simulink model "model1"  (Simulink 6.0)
settings: Solver=ode1  StartTime=0.0  StopTime=3.0  FixedStep=0.001  RelTol=1e-3
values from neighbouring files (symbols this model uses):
  a = 0.001    [slpriv1m.m]    (also in red1m.m; SAUAnalizeProject.m = axes( 'Parent',  centerPanel,   'Projection', 'perspective',; TESTm.m)
  ak0 = 1    [slpriv1m.m]    (also in TESTm.m)
  ak1 = 0.5    [slpriv1m.m]    (also in TESTm.m)
  ap0 = 1    [slpriv1m.m]    (also in TESTm.m)
  ap1 = 0.001    [slpriv1m.m]    (also in TESTm.m)
  bk0 = 0    [slpriv1m.m]    (also in TESTm.m)
  bk1 = 0.5    [slpriv1m.m]    (also in TESTm.m)
  bp0 = 1    [slpriv1m.m]    (also in TESTm.m)
  bp1 = 0.001    [slpriv1m.m]    (also in TESTm.m)
  c = 2000000    [slpriv1m.m]    (also in red1m.m; TESTm.m)
  F1 = 0    [slpriv1m.m]    (also in main5.m = peaks(35); main7.m = zeros(A1n,A2n); red1m.m; TESTm.m)
  F2 = 0    [slpriv1m.m]    (also in main5.m = membrane; main7.m = zeros(A1n,A2n); red1m.m; TESTm.m)
  G1 = 0    [slpriv1m.m]    (also in red1m.m; TESTm.m)
  G2 = 0    [slpriv1m.m]    (also in red1m.m; TESTm.m)
  i = 100    [slpriv1m.m]    (also in red1m.m; SAUAnalizeProject.m = find( isoLevel == src ); TESTm.m)
  J = 0.04    [slpriv1m.m]    (also in TESTm.m)
  Jn = 200    [slpriv1m.m]    (also in red1m.m; TESTm.m)
  k1 = 1/R    (= 2)    [myparam.m]    (also in slpriv1m.m; TESTm.m)
  K1 = 3    [dz.m]    (also in fun_F6.m = A2; fun_F7.m = A2; fun_F9.m = A1m1(i); main7.m = 0.5)
  K2 = 2    [dz.m]    (also in fun_F6.m = A1; fun_F7.m = A1; fun_F9.m = A2m1(j); main7.m = 0.5)
  K3 = 0    [dz.m]    (also in fun_F6.m = A1; fun_F7.m = A1; fun_F9.m = A3m1(k); main7.m = 0.5)
  Kc = 0.0015    [slpriv1m.m]    (also in TESTm.m)
  Ki = 0.0003    [slpriv1m.m]    (also in TESTm.m)
  Kk = 22500    [slpriv1m.m]    (also in TESTm.m)
  km = 0.36    [myparam.m]    (also in slpriv1m.m; TESTm.m)
  kv = 0.45    [myparam.m]    (also in slpriv1m.m; TESTm.m)
  T = L/R    (= 0.02)    [myparam.m]    (also in slpriv1m.m; TESTm.m)

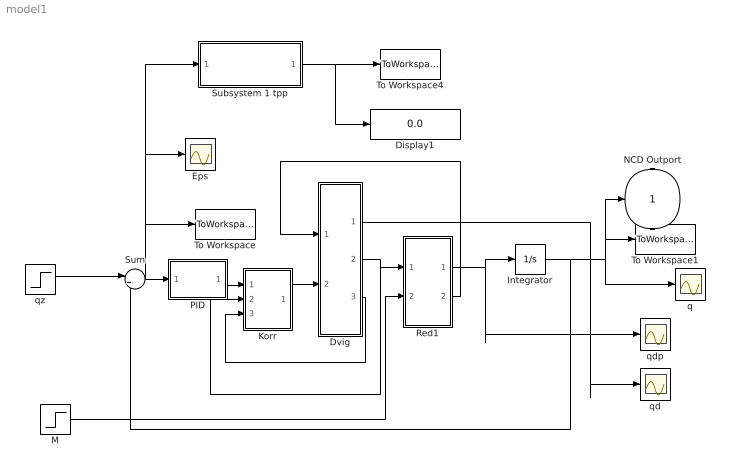
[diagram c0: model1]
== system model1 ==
  Display1 : Display
  Dvig : Subsystem  AncestorBlock=simulink3/Signals & Systems/SubSystem
  Eps : Scope
  Integrator : Integrator
  Korr : Subsystem
  M : Step  Time=0  After=0  SampleTime=0
  PID : Subsystem
  Red1 : Subsystem
  Subsystem 1 tpp : Subsystem
  Sum : Sum  Inputs=|+-
  To Workspace : ToWorkspace  VariableName=simouteps  SampleTime=-1  SaveFormat=Structure
  To Workspace1 : ToWorkspace  VariableName=simoutq  SampleTime=-1  SaveFormat=Structure
  To Workspace4 : ToWorkspace  VariableName=tpptek  SampleTime=-1  SaveFormat=Array
  q : Scope
  qd : Scope
  qdp : Scope
  qz : Step  Time=0  After=0.1  SampleTime=0
  NCD Outport : Outport  InitialOutput=0
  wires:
  Sum/1 -> PID/1(eps), To Workspace/1, Eps/1, Subsystem 1 tpp/1(In1:Signal)
  PID/1(ueps) -> Korr/1(u_eps)
  Red1/2(M2M) -> Dvig/1(Mv)
  Korr/1(u_d) -> Dvig/2(u)
  Dvig/2(qd') -> Red1/1(q1p), Korr/2(qdp)
  Dvig/3(ia) -> Korr/3(ia)
  M/1 -> Red1/2(-M2)
  Red1/1(q2p) -> Integrator/1, qdp/1
  Integrator/1 -> Sum/2, To Workspace1/1, NCD Outport/1, q/1
  Dvig/1(qd) -> qd/1
  Subsystem 1 tpp/1(Out1:tpp) -> To Workspace4/1, Display1/1
  qz/1 -> Sum/1

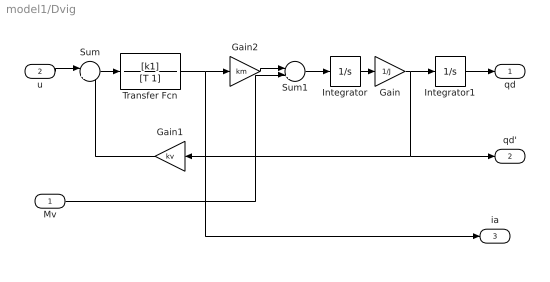
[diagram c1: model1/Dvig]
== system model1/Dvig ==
  Mv : Inport  Port=1  LatchInput=off
  u : Inport  Port=2  LatchInput=off
  Gain : Gain  Gain=1/J
  Gain1 : Gain  Orientation=left  Gain=kv
  Gain2 : Gain  Gain=km
  Integrator : Integrator
  Integrator1 : Integrator
  Sum : Sum  Inputs=|+-
  Sum1 : Sum  Inputs=|++
  Transfer Fcn : TransferFcn  Numerator=[k1]  Denominator=[T 1]
  qd : Outport
  qd' : Outport  Port=2
  ia : Outport  Port=3
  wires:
  u/1 -> Sum/1
  Gain1/1 -> Sum/2
  Sum/1 -> Transfer Fcn/1
  Transfer Fcn/1 -> Gain2/1, ia/1
  Gain2/1 -> Sum1/1
  Mv/1 -> Sum1/2
  Sum1/1 -> Integrator/1
  Integrator/1 -> Gain/1
  Gain/1 -> Integrator1/1, Gain1/1, qd'/1
  Integrator1/1 -> qd/1

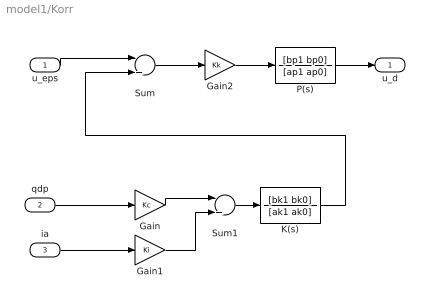
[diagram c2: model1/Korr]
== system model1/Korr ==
  u_eps : Inport  Port=1  LatchInput=off
  qdp : Inport  Port=2  LatchInput=off
  ia : Inport  Port=3  LatchInput=off
  Gain : Gain  Gain=Kc
  Gain1 : Gain  Gain=Ki
  Gain2 : Gain  Gain=Kk
  K(s) : TransferFcn  Numerator=[bk1 bk0]  Denominator=[ak1 ak0]
  P(s) : TransferFcn  Numerator=[bp1 bp0]  Denominator=[ap1 ap0]
  Sum : Sum  Inputs=|+-
  Sum1 : Sum  Inputs=|++
  u_d : Outport
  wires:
  u_eps/1 -> Sum/1
  qdp/1 -> Gain/1
  ia/1 -> Gain1/1
  Sum/1 -> Gain2/1
  Gain/1 -> Sum1/1
  Gain1/1 -> Sum1/2
  Gain2/1 -> P(s)/1
  P(s)/1 -> u_d/1
  Sum1/1 -> K(s)/1
  K(s)/1 -> Sum/2

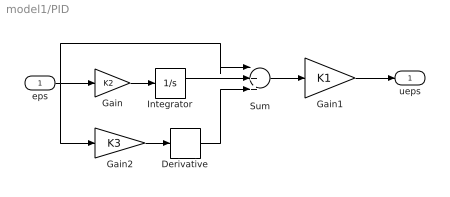
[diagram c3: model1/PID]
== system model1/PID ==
  eps : Inport  Port=1  LatchInput=off
  Derivative : Derivative
  Gain : Gain  Gain=K2
  Gain1 : Gain  Gain=K1
  Gain2 : Gain  Gain=K3
  Integrator : Integrator
  Sum : Sum  Inputs=|+++
  ueps : Outport
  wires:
  Gain1/1 -> ueps/1
  Sum/1 -> Gain1/1
  Gain/1 -> Integrator/1
  eps/1 -> Gain/1, Sum/1, Gain2/1
  Integrator/1 -> Sum/2
  Gain2/1 -> Derivative/1
  Derivative/1 -> Sum/3

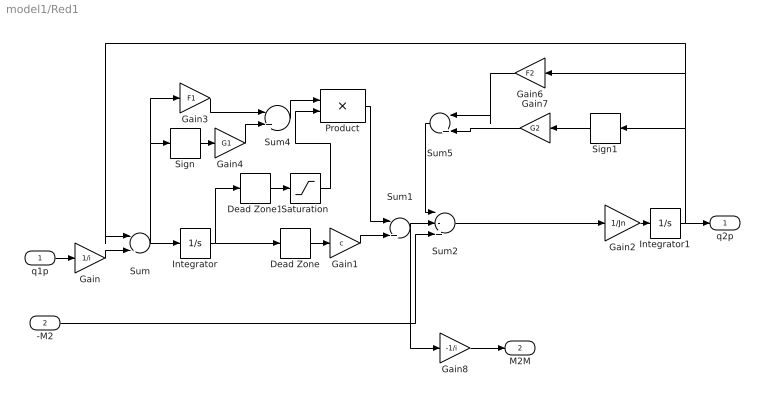
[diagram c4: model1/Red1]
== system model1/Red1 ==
  q1p : Inport  Port=1  LatchInput=off
  -M2 : Inport  Port=2  LatchInput=off
  Dead Zone : DeadZone  LowerValue=-a  UpperValue=a
  Dead Zone1 : DeadZone  LowerValue=-a  UpperValue=a
  Gain : Gain  Gain=1/i
  Gain1 : Gain  Gain=c
  Gain2 : Gain  Gain=1/Jn
  Gain3 : Gain  Gain=F1
  Gain4 : Gain  Gain=G1
  Gain6 : Gain  Orientation=left  Gain=F2
  Gain7 : Gain  Orientation=left  Gain=G2
  Gain8 : Gain  Gain=-1/i
  Integrator : Integrator
  Integrator1 : Integrator
  Product : Product
  Saturation : Saturate  UpperLimit=a  LowerLimit=-a
  Sign : Signum
  Sign1 : Signum  Orientation=left
  Sum : Sum  Inputs=|-+
  Sum1 : Sum  Inputs=|++
  Sum2 : Sum  Inputs=|-++
  Sum4 : Sum  Inputs=|++
  Sum5 : Sum  Orientation=left  Inputs=|++
  q2p : Outport
  M2M : Outport  Port=2
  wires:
  q1p/1 -> Gain/1
  Gain/1 -> Sum/2
  Sum/1 -> Integrator/1, Gain3/1, Sign/1
  Integrator/1 -> Dead Zone/1, Dead Zone1/1
  Dead Zone/1 -> Gain1/1
  Gain1/1 -> Sum1/2
  Sum1/1 -> Sum2/2, Gain8/1
  Sum2/1 -> Gain2/1
  Gain2/1 -> Integrator1/1
  Integrator1/1 -> q2p/1, Sign1/1, Gain6/1, Sum/1
  -M2/1 -> Sum2/3
  Gain3/1 -> Sum4/1
  Gain4/1 -> Sum4/2
  Sign/1 -> Gain4/1
  Sum4/1 -> Product/1
  Product/1 -> Sum1/1
  Sum5/1 -> Sum2/1
  Gain6/1 -> Sum5/1
  Gain7/1 -> Sum5/2
  Sign1/1 -> Gain7/1
  Gain8/1 -> M2M/1
  Dead Zone1/1 -> Saturation/1
  Saturation/1 -> Product/2

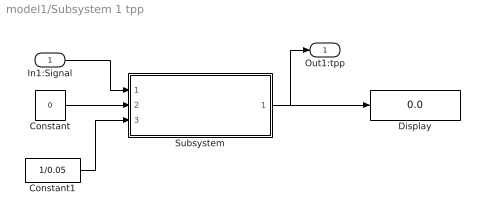
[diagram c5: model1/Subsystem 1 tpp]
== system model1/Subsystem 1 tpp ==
  In1:Signal : Inport  Port=1  LatchInput=off
  Constant : Constant  Value=0
  Constant1 : Constant  Value=1/0.05
  Display : Display
  Subsystem : Subsystem
  Out1:tpp : Outport
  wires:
  In1:Signal/1 -> Subsystem/1(In1:Signal)
  Constant/1 -> Subsystem/2(In2:ustzn)
  Constant1/1 -> Subsystem/3(In3:Lavel)
  Subsystem/1(Out1) -> Display/1, Out1:tpp/1

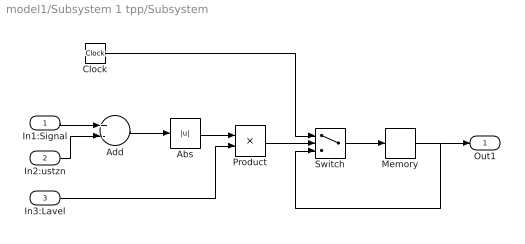
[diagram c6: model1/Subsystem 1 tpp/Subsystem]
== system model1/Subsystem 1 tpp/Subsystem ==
  In1:Signal : Inport  Port=1  LatchInput=off
  In2:ustzn : Inport  Port=2  LatchInput=off
  In3:Lavel : Inport  Port=3  LatchInput=off
  Abs : Abs
  Add : Sum  Inputs=+-  OutScaling=2^-10
  Clock : Clock
  Memory : Memory
  Product : Product
  Switch : Switch  Threshold=1
  Out1 : Outport
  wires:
  In1:Signal/1 -> Add/1
  In2:ustzn/1 -> Add/2
  Add/1 -> Abs/1
  Abs/1 -> Product/1
  In3:Lavel/1 -> Product/2
  Product/1 -> Switch/2
  Clock/1 -> Switch/1
  Switch/1 -> Memory/1
  Memory/1 -> Out1/1, Switch/3
